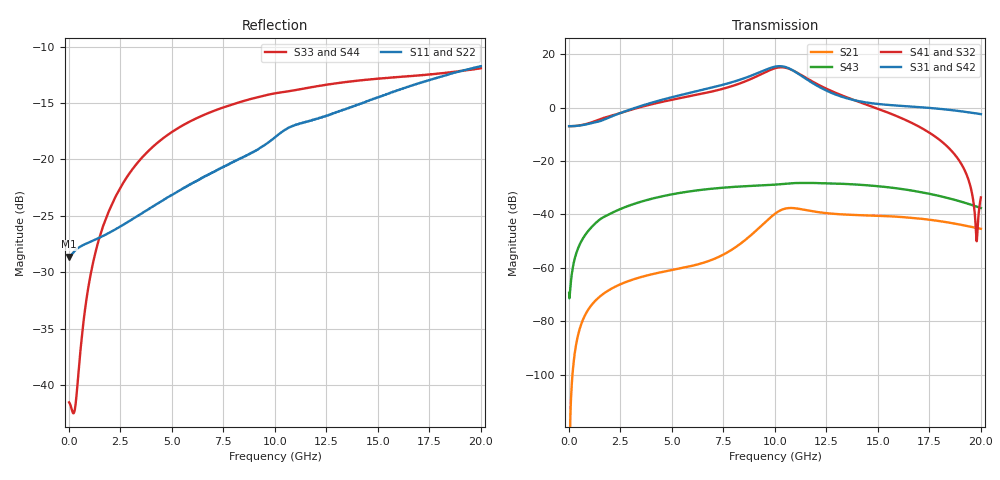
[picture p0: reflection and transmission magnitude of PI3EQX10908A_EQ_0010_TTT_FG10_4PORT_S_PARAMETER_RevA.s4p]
! NPort=4 DATA=2000 NOISE=0 GROUPDELAY=0 COMPLEX_DATAFORMAT=POLAR
! NumOfBlock=1 NumOfParam=0
! .MODEL Smodel S TSTONEFILE=PI3EQX10908A_EQ_0010_TTT_FG10_4PORT_S_PARAMETER_RevA.s4p TYPE=S
!  -- The above .MODEL line can be used for the S element in the netlist.
! The s parameter is extracted from the linear redriver, it is not bi-directional; only s(4,1)s(4,2) and s(3,1)s(3,2)
! should be the insertion loss
!Port definition:
!Port1 = input+
!Port2 = input-
!Port3 = output+
!Port4 = output-
# Hz S MA R  50
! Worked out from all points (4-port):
!   2000 points, 10 MHz to 20 GHz, reference 50 ohm
!   strongest paths, dB at 10 MHz, 5.01 GHz, 10.01 GHz, 15.01 GHz, 20 GHz:
!     S31: -6.9, 3.9, 15.4, 1.4, -2.4
!     S42: -6.9, 3.9, 15.4, 1.4, -2.4
!     S41: -6.9, 3.0, 14.8, -0.4, -33.6
!     S32: -6.9, 3.0, 14.8, -0.5, -33.6
!     S43: -69.4, -32.4, -28.8, -29.4, -37.6
!     S21: -127.3, -60.8, -39.7, -40.5, -45.4
!   lowest |S11| = -28.6 dB at 10 MHz (marker M1), VSWR 1.08, Z = 46.4 - j0.024 ohm
!   |S11| at or under -10 dB: start of sweep to end of sweep
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1e7  0.03701 -179.6  4.328e-07 13.5  0 0.0  0 0.0
     4.328e-07 13.5  0.03701 -179.6  0 0.0  0 0.0
     0.4502 -0.0  0.4502 180.0  0.008374 26.0  0.00034 -27.1
     0.4502 180.0  0.4502 -0.0  0.00034 -27.1  0.008374 26.0
7.69e9  0.09441 -117.9  0.001947 129.3  9.289e-07 54.5  3.681e-07 132.6
        0.001947 129.3  0.09444 -117.9  3.681e-07 132.6  9.289e-07 54.5
        2.827 -49.5  2.381 123.6  0.1726 4.0  0.03219 6.1
        2.381 123.6  2.827 -49.5  0.03219 6.1  0.1726 4.0
9.79e9  0.1211 -110.6  0.008851 119.6  4.666e-06 6.2  2.887e-06 122.8
        0.008851 119.6  0.1211 -110.6  2.887e-06 122.8  4.666e-06 6.2
        5.551 -108.5  5.11 66.2  0.1949 -11.4  0.03569 -14.2
        5.11 66.2  5.551 -108.5  0.03569 -14.2  0.1949 -11.4
1.061e10  0.1374 -111.1  0.0131 81.4  5.953e-06 -28.1  6.353e-06 85.0
          0.0131 81.4  0.1374 -111.1  6.353e-06 85.0  5.953e-06 -28.1
          5.592 -156.2  5.471 16.6  0.2005 -16.7  0.03801 -22.6
          5.471 16.6  5.592 -156.2  0.03801 -22.6  0.2005 -16.7
1.176e10  0.149 -112.6  0.0116 42.6  5.751e-06 -35.4  9.644e-06 39.7
          0.0116 42.6  0.149 -112.6  9.644e-06 39.7  5.751e-06 -35.4
          2.998 160.2  3.177 -33.6  0.2092 -23.0  0.0389 -37.6
          3.177 -33.6  2.998 160.2  0.0389 -37.6  0.2092 -23.0
1.47e10  0.1843 -110.7  0.009538 4.4  2.227e-05 -53.3  2.42e-05 -25.1
         0.009539 4.4  0.1844 -110.7  2.42e-05 -25.1  2.227e-05 -53.3
         1.209 134.8  1.05 -91.8  0.227 -37.4  0.03463 -73.7
         1.05 -91.8  1.209 134.8  0.03463 -73.7  0.227 -37.4
2e10  0.2594 -114.0  0.005385 -47.4  9.198e-05 -147.8  7.23e-05 -136.8
      0.005385 -47.4  0.2595 -114.0  7.23e-05 -136.8  9.198e-05 -147.8
      0.7562 62.7  0.0209 -20.5  0.254 -52.2  0.01317 -136.8
      0.02089 -20.5  0.7561 62.7  0.01317 -136.8  0.254 -52.2
